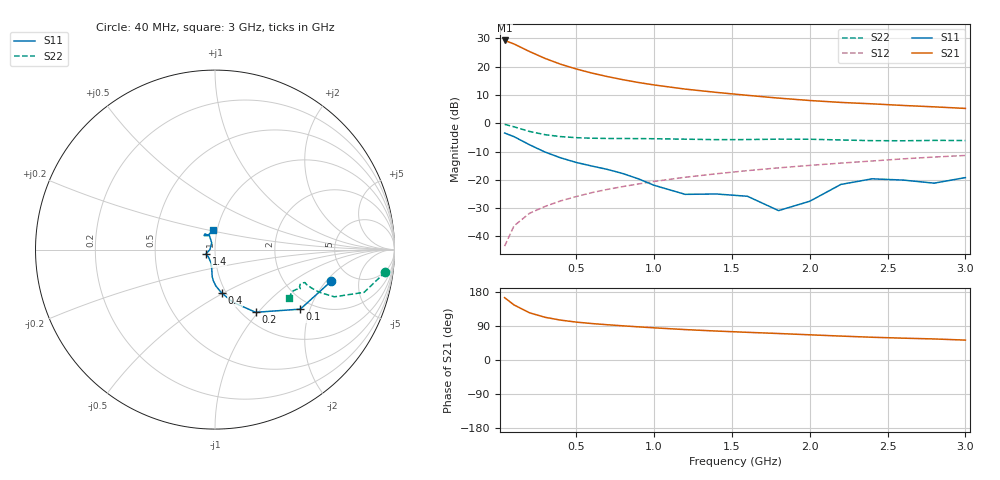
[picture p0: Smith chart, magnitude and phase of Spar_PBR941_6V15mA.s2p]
! Filename:  PBR941O.S2P  Version:  3.0
! NXP part #:  PBR941  Date: July 1998
! Bias condition:  Vce=6V, Ic=15mA
#  MHz  S  MA  R 50
! Freq  S11  S21  S12  S22
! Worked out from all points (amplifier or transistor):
!   21 points, 40 MHz to 3 GHz, reference 50 ohm
!   highest |S21| = 29.3 dB at 40 MHz (marker M1)
!   |S21| within 3 dB of that: start of sweep to 165.9 MHz
!   unconditionally stable (mu >= 1): 878.7 MHz to 2.29 GHz
!   at 300 MHz: K = 0.79, MSG = 26.2 dB, |S12| = -29.4 dB
!   at 1 GHz: K = 1.01, MAG = 16.4 dB, |S12| = -20.6 dB
!   at 3 GHz: K = 0.98, MSG = 8.3 dB, |S12| = -11.4 dB
!   lowest NFmin = 2.00 dB at 900 MHz
!   S11 on the Smith chart (normalised r, x): 40 MHz: 3.54, -2.27; 100 MHz: 1.72, -1.72; 200 MHz: 1.15, -0.97; 400 MHz: 0.95, -0.49; 1.4 GHz: 0.90, -0.04; 3 GHz: 0.95, +0.21
40  0.6708 -15.2  29.04 164.5  0.006709 82.7  0.9569 -7.5
100  0.5794 -34.9  25.2 145.4  0.01528 76.9  0.8644 -16.0
200  0.4163 -57.1  18.5 124.6  0.02559 71.9  0.7152 -21.6
300  0.309 -71.3  13.98 112.7  0.03385 72.3  0.6271 -22.2
400  0.2444 -81.2  11.04 105.2  0.04238 73.3  0.5802 -21.7
500  0.2027 -88.6  9.097 100.0  0.05051 75.1  0.5554 -21.2
600  0.1751 -92.9  7.707 96.2  0.05929 76.0  0.5431 -20.7
700  0.1528 -95.8  6.68 93.1  0.0676 77.2  0.5381 -20.4
800  0.1289 -97.6  5.878 90.2  0.07588 77.6  0.5371 -20.3
900  0.1038 -100.0  5.247 87.5  0.08453 77.9  0.5349 -20.2
1000  0.08004 -104.7  4.75 84.9  0.09347 78.0  0.532 -20.2
1200  0.05528 -132.0  4.011 80.3  0.1109 78.0  0.5221 -20.8
1400  0.05612 -154.0  3.509 76.4  0.1278 77.8  0.5124 -22.2
1600  0.05115 -156.4  3.112 73.1  0.1452 77.8  0.5144 -23.6
1800  0.02853 -179.3  2.778 69.9  0.1625 77.5  0.5226 -24.6
2000  0.04172 115.8  2.521 66.5  0.1796 76.8  0.521 -25.1
2200  0.08276 112.0  2.332 63.1  0.1973 75.8  0.5057 -25.9
2400  0.104 122.6  2.202 60.0  0.2149 75.3  0.4919 -27.9
2600  0.09888 128.0  2.06 57.6  0.2344 74.9  0.4897 -30.6
2800  0.08722 117.0  1.947 55.5  0.2526 74.2  0.4971 -32.4
3000  0.1094 96.0  1.827 52.5  0.2692 73.1  0.494 -32.9
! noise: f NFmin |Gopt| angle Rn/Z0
500  2.017  0.148  12.9  0.263
900  2.003  0.06  -23.43  0.197
1000  2.059  0.081  27.92  0.261
2000  2.623  0.131  -127.3  0.297
